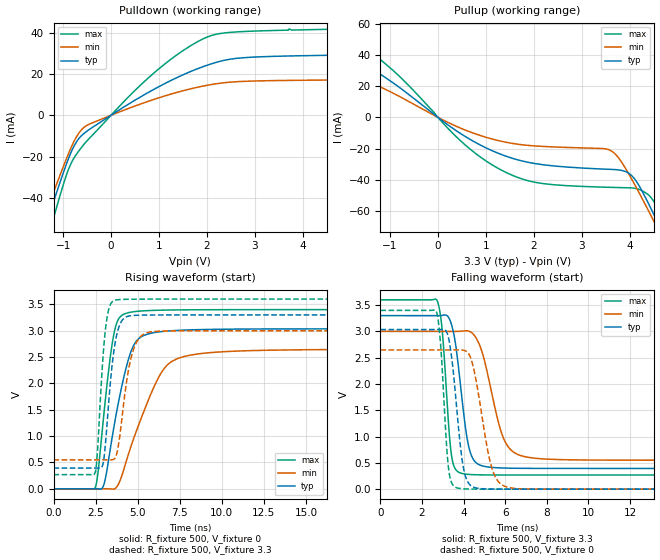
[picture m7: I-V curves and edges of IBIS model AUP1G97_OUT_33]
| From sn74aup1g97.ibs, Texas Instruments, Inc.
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[Model]   AUP1G97_OUT_33
Model_type  Output
Vref =   0
Rref =   1E6
Cref =   30p
Vmeas =   1.65
| variable   typ   min   max
C_comp   2.73pF   1.81pF   4.12pF
| C_pullup   3.12pF   1.81pF   4.12pF
| C_pulldown   2.33pF   2.13pF   2.90pF
[Temperature Range]   40   100   -40
| Ambient temperature   25   85   -40
[Voltage range]   3.3   3   3.6
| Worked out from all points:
|   slope of the pulldown table from 0 to 0.495 V, typ, clamps not added: 68.4 ohm
|   slope of the pullup table from 0 to 0.495 V, typ, clamps not added: 45.8 ohm
|   rising waveform, R_fixture 500, V_fixture 0: 20-80 % time 1.13ns typ, 1.92ns min, 706ps max; typ from 0 V to 3.04 V
|   falling waveform, R_fixture 500, V_fixture 3.3: 20-80 % time 538ps typ, 889ps min, 346ps max; typ from 3.3 V to 0.394 V
|   rising waveform, R_fixture 500, V_fixture 3.3: 20-80 % time 517ps typ, 676ps min, 401ps max; typ from 0.394 V to 3.3 V
|   falling waveform, R_fixture 500, V_fixture 0: 20-80 % time 463ps typ, 698ps min, 310ps max; typ from 3.04 V to 0 V
[Pulldown]
| AUP1G97_OUT_33
|   Voltage   I(typ)   I(min)   I(max)
-3.6V     -218.7mA   -196.3mA   -248.6mA
-1.515V   -64.37mA   -57.31mA   -75.82mA
-1.39V    -55.35mA   -49.29mA   -65.41mA
-1.275V   -47.14mA   -42mA      -55.89mA
-870mV    -19.93mA   -17.62mA   -25.18mA
-720mV    -12.85mA   -10.38mA   -18.82mA
-545mV    -8.444mA   -5.509mA   -13.51mA
940mV     13.13mA    8.018mA    21.36mA
1.5V      19.56mA    11.86mA    31.27mA
2.045V    24.53mA    14.67mA    38.2mA
3.1V      28.27mA    16.63mA    40.81mA
7.2V      29.73mA    17.36mA    42.67mA
[Pullup]
| AUP1G97_OUT_33
|   Voltage   I(typ)   I(min)   I(max)
-3.6V     42.88mA    27.27mA    57.92mA
-2.465V   31.53mA    19.52mA    45.85mA
-1.53V    32.87mA    22.09mA    44.95mA
-755mV    18.1mA     12.64mA    24.89mA
555mV     -11.98mA   -7.942mA   -17.3mA
1.65V     -27.07mA   -17.13mA   -38.31mA
3.61V     -33.32mA   -21.39mA   -44.82mA
4.08V     -38.63mA   -41.77mA   -45.28mA
4.375V    -54.25mA   -58.9mA    -49.24mA
4.565V    -66.24mA   -70.37mA   -57.33mA
4.775V    -80.02mA   -83.29mA   -71.37mA
7.2V      -250.7mA   -240.9mA   -257mA
[Ramp]
| AUP1G97_OUT_33
| variable   typ   min   max
dV/dt_r   1.82/1.13E-09   1.59/1.93E-09   2.04/7.08E-10
dV/dt_f   1.75/5.45E-10   1.48/8.94E-10   2.01/3.51E-10
R_load = 500
[Rising Waveform]
| AUP1G97_OUT_33
R_fixture =   500
C_fixture =   0
L_fixture =   0
V_fixture =   0
V_fixture_min = 0
V_fixture_max = 0
|   Time   V(typ)   V(min)   V(max)
0s        24.73nV    82.54nV    2.123nV
2.5ns     455.8uV    1.777uV    41.63mV
2.995ns   84.91mV    558.2uV    1.427V
3.54ns    1.084V     -6.3mV     2.857V
3.825ns   1.588V     70.01mV    3.2V
4.29ns    2.267V     490.9mV    3.327V
4.965ns   2.819V     1.133V     3.367V
6.275ns   2.977V     2.133V     3.388V
7.77ns    3.012V     2.512V     3.395V
30.7ns    3.035V     2.647V     3.399V
[Falling Waveform]
| AUP1G97_OUT_33
R_fixture =   500
C_fixture =   0
L_fixture =   0
V_fixture =   3.3
V_fixture_min = 3
V_fixture_max = 3.6
|   Time   V(typ)   V(min)   V(max)
0s        3.3V       3V         3.6V
2.74ns    3.3V       3V         3.575V
2.97ns    3.305V     3V         3.025V
3.41ns    3.14V      2.999V     666.5mV
3.885ns   1.853V     3.004V     302.1mV
4.2ns     896.7mV    3.009V     282.3mV
4.53ns    531.9mV    2.917V     275mV
5.91ns    402.1mV    976.3mV    269.6mV
6.915ns   396.1mV    620.6mV    269.3mV
30.7ns    394.1mV    550mV      269.3mV
[Rising Waveform]
| AUP1G97_OUT_33
R_fixture =   500
C_fixture =   0
L_fixture =   0
V_fixture =   3.3
V_fixture_min = 3
V_fixture_max = 3.6
|   Time   V(typ)   V(min)   V(max)
0s        394.1mV    550mV      269.3mV
2.475ns   394.3mV    550.1mV    314.2mV
2.615ns   394.3mV    550.2mV    737.1mV
2.89ns    426.2mV    550.3mV    2.27V
3.08ns    836.9mV    550.1mV    3.012V
3.61ns    2.669V     568.7mV    3.575V
4ns       3.156V     1.164V     3.592V
4.635ns   3.286V     2.52V      3.597V
5.595ns   3.296V     2.966V     3.599V
30.7ns    3.3V       3V         3.6V
[Falling Waveform]
| AUP1G97_OUT_33
R_fixture =   500
C_fixture =   0
L_fixture =   0
V_fixture =   0
V_fixture_min = 0
V_fixture_max = 0
|   Time   V(typ)   V(min)   V(max)
0s        3.035V     2.647V     3.399V
2.7ns     3.035V     2.647V     3.367V
2.9ns     3.036V     2.647V     2.716V
3.275ns   2.879V     2.648V     398.5mV
3.705ns   1.379V     2.649V     21.75mV
3.96ns    476.7mV    2.644V     8.162mV
4.235ns   114.8mV    2.579V     3.353mV
5.345ns   2.469mV    420.2mV    151.8uV
6.125ns   446.5uV    34.94mV    28.59uV
30.7ns    -26.93nV   58.34nV    -26.55nV
